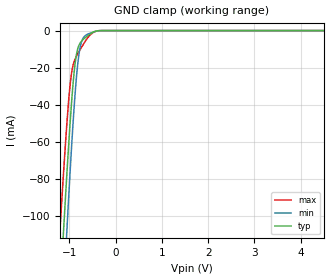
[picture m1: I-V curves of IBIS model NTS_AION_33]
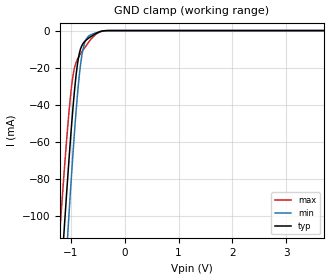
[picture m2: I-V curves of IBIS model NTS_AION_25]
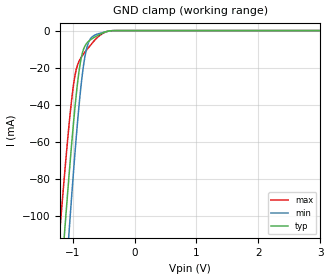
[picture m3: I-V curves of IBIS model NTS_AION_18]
| NXP Semiconductors
| Logic Products Group
| IBIS model of NTS0101
| SINGLE, DUAL-SUPPLY VOLTAGE-LEVEL TRANSLATING AUTO-DIRECTION SENSING
| TRANSCEIVER WITH OPEN-DRAIN OUTPUTS (3-STATE OE)
|[Packages]:
|[Package1]: SC88 (GW) 6-pin Package
|[Package2]: TSSOP6 (GV) 6-pins package
|[Package3]: XSON6 (GM) 6-pins package
|[Package4]: XSON6 (GF) 6-pins package
|[Package5]: XSON6 (GS) 6-pins package
[IBIS Ver]   3.2
[File Name]   nts0101.ibs
[File Rev]   1.0
[Date]   20-May-2011
[Source]   File created from simulations by LPG
   NXP Semiconductors Nijmegen
[Notes]   V1.0   Ibis model.
   Revision History
   Version Date   Author/Editor   Description
   1.0   May 2011   RRV   Initial Model
   Remarks: - The Power Clamp curves have been omitted from the input
   since there is no power clamp diode.
   - IBISCHK 5.0.3 used
[Disclaimer]
   NXP Semiconductors warrants and represents that the IBIS model
   identified herein is owned by NXP Semiconductors (NXP). The
   model provided is not warranted as fully representing all of the
   operating characteristics and specifications of the semiconductor
   products to which the model relates.  Moreover, unless there is a
   signed, written agreement to the contrary, this IBIS model is
   furnished on an "as is" basis without support or warranty of any
   kind, either expressed or implied, regarding the use thereof, and
   NXP specifically disclaims all implied warranties of
   merchantability and fitness of the model for any purpose.
   NXP does not assume any liability arising out of the application
   or use of this IBIS model including infringement of patents and
   copyrights, nor does NXP convey any license under its patents and
   copyrights or the rights of others.
   NXP provides IBIS models as a service to our customers. You and
   your company shall not distribute, convey, sell, or give these models
   to anyone else without receiving prior written permission from
   NXP.
   NXP reserves the right to make changes without notice to these
   IBIS models to improve reliability, function, or design.
   Please be aware that your receipt and subsequent use of the IBIS
   information provided shall serve as acceptance of the terms and
   conditions of this agreement.  If you do not accept these terms,
   you should return or destroy the IBIS models and any other
   accompanying information immediately.
[Copyright]
   (C) Copyright 2011 NXP Semiconductors
   All rights reserved
|   Info for  SC88 (GW) 6-pin Package
[Component]   NTS0101_GW
[Manufacturer]   NXP Semiconductors
[package]
|   typ   min   max
R_pkg  3.9397E-02  2.6064E-02  5.8029E-02
L_pkg  9.0534E-10  7.0046E-10  1.1872E-09
C_pkg  1.8035E-13  1.2290E-13  3.5012E-13
[Pin] signal_name   model_name   R_pin   L_pin   C_pin
   1   VDDA   POWER 3.0056E-02 7.6713E-10 1.2290E-13
   2   GND   GND 2.6064E-02 7.0046E-10 3.5012E-13
   3   A   NTS_AION 5.0072E-02 1.0663E-09 1.4645E-13
   4   B   NTS_BION 5.8029E-02 1.1872E-09 1.6820E-13
   5   OE   NTS_CTRLIN 3.4118E-02 8.2339E-10 1.5073E-13
   6   VDDB   POWER 3.8045E-02 8.8757E-10 1.4368E-13
|   Info for  TSSOP6 (GV) 6-pins package
[Component]   NTS0101_GV
[Manufacturer]   NXP Semiconductors
[Package]
|   Typ   Min   Max
R_pkg   8.223E-02   8.127E-02   8.329E-02
L_pkg   1.527E-09   1.437E-09   1.626E-09
C_pkg   2.754E-13   2.307E-13   4.138E-13
[Pin] signal_name   model_name   R_pin   L_pin   C_pin
   1   VDDA   POWER 8.329E-02 1.622E-09 2.613E-13
   2   GND   GND 8.127E-02 1.437E-09 4.138E-13
   3   A   NTS_AION 8.324E-02 1.626E-09 2.540E-13
   4   B   NTS_BION 8.183E-02 1.491E-09 2.307E-13
   5   OE   NTS_CTRLIN 8.187E-02 1.489E-09 2.619E-13
   6   VDDB   POWER 8.320E-02 1.613E-09 2.601E-13
|   Info for  XSON6 (GM) 6-pins package
[Component]   NTS0101_GM
[Manufacturer]   NXP Semiconductors
[Package]
|   Typ   Min   Max
R_pkg   3.997E-02   3.996E-02   3.998E-02
L_pkg   6.173E-10   6.152E-10   6.184E-10
C_pkg   1.884E-13   1.795E-13   2.057E-13
[Pin] signal_name   model_name   R_pin   L_pin   C_pin
   1   VDDA   POWER 3.997E-02 6.184E-10 1.801E-13
   2   GND   GND 3.996E-02 6.152E-10 2.057E-13
   3   A   NTS_AION 3.997E-02 6.182E-10 1.795E-13
   4   B   NTS_BION 3.998E-02 6.184E-10 1.795E-13
   5   OE   NTS_CTRLIN 3.997E-02 6.154E-10 2.057E-13
   6   VDDB   POWER 3.997E-02 6.179E-10 1.798E-13
|   Info for  XSON6 (GF) 6-pins package
[Component]   NTS0101_GF
[Manufacturer]   NXP Semiconductors
[Package]
|   Typ   Min   Max
R_pkg   3.978E-02   3.977E-02   3.979E-02
L_pkg   6.070E-10   6.066E-10   6.077E-10
C_pkg   1.209E-13   1.153E-13   1.316E-13
[Pin] signal_name   model_name   R_pin   L_pin   C_pin
   1   VDDA   POWER 3.979E-02 6.077E-10 1.160E-13
   2   GND   GND 3.979E-02 6.071E-10 1.316E-13
   3   A   NTS_AION 3.978E-02 6.072E-10 1.153E-13
   4   B   NTS_BION 3.977E-02 6.067E-10 1.153E-13
   5   OE   NTS_CTRLIN 3.978E-02 6.066E-10 1.315E-13
   6   VDDB   POWER 3.978E-02 6.069E-10 1.155E-13
|   Info for  XSON6 (GS) 6-pins package
[Component]   NTS0101_GS
[Manufacturer]   NXP Semiconductors
[Package]
|   Typ   Min   Max
R_pkg   3.5879E-02   3.5869E-02   3.5886E-02
L_pkg   4.5703E-10   4.5658E-10   4.5769E-10
C_pkg   1.1638E-13   1.1080E-13   1.2708E-13
[Pin] signal_name   model_name   R_pin   L_pin   C_pin
   1   VDDA   POWER 3.5886E-02 4.5769E-10 1.1155E-13
   2   GND   GND 3.5886E-02 4.5710E-10 1.2708E-13
   3   A   NTS_AION 3.5877E-02 4.5721E-10 1.1080E-13
   4   B   NTS_BION 3.5869E-02 4.5673E-10 1.1080E-13
   5   OE   NTS_CTRLIN 3.5878E-02 4.5658E-10 1.2704E-13
   6   VDDB   POWER 3.5879E-02 4.5686E-10 1.1098E-13
[Model Selector]   NTS_AION
NTS_AION_33   3.3V Vcc I/O model, non-inverting
NTS_AION_25   2.5V Vcc I/O model, non-inverting
NTS_AION_18   1.8V Vcc I/O model, non-inverting
[Model Selector]   NTS_BION
NTS_BION_50   5.0V Vcc I/O model, non-inverting
NTS_BION_33   3.3V Vcc I/O model, non-inverting
NTS_BION_25   2.5V Vcc I/O model, non-inverting
[Model Selector]   NTS_CTRLIN
NTS_CTRLIN_33   3.3V Vcc Input model
NTS_CTRLIN_25   2.5V Vcc Input model
NTS_CTRLIN_18   1.8V Vcc Input model
| Models and submodels in the file (9): NTS_AION_33 (Input), NTS_AION_25 (Input), NTS_AION_18 (Input), NTS_BION_50 (Input), NTS_BION_33 (Input), NTS_BION_25 (Input), NTS_CTRLIN_33 (Input), NTS_CTRLIN_25 (Input), NTS_CTRLIN_18 (Input)
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| Remark: If your software does not support the Model Selector
|   Please comment out the lines of the Model Selector, which
|   contain the name of the Model, except the one you want to use.
|   Model NTS_AION_33
[Model]   NTS_AION_33
Model_type   Input
Vinh  =  2.9
Vinl  =  0.15
C_comp   1.9335pF   1.4778pF   2.7541pF
[Model Spec]
| Note: The input and output voltage ratings may be exceeded if the input and
|   output current ratings are observed (please refer to the data sheet)
|   Subparameter   typ   min   max
Vinh   2.9   2.6   3.2
Vinl   0.15   0.15   0.15
| Overshoot
S_overshoot_high   6.5   6.5   6.5   | Static overshoot
S_overshoot_low   -0.5   -0.5   -0.5
D_overshoot_high   7.2   7.2   7.2   | Dynamic overshoot
D_overshoot_low   -1.0   -1.0   -1.0
D_overshoot_time   3n   3n   3n
|Ambient temperature:   25   85   -40
[Temperature Range]   40   100   -25
[Voltage Range]   3.3   3.0   3.6
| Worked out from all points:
|   GND clamp passes 1 mA (typ) near -0.50 V on its own axis
|Process Range   nominal   slow   fast
[GND_clamp]
|   voltage   I(typ)   I(min)   I(max)
-5.5V     -2.251A    -2.513A    -2.036A
-1.2V     -140.4mA   -178.4mA   -105.8mA
-1.12V    -105mA     -138.9mA   -74.04mA
-1.06V    -79.44mA   -110.2mA   -51.97mA
-1V       -55.52mA   -82.82mA   -33.13mA
-960mV    -41.02mA   -65.56mA   -24.03mA
-880mV    -18.45mA   -35.09mA   -15.56mA
-820mV    -9.803mA   -18.09mA   -12.49mA
-740mV    -5.756mA   -6.204mA   -9.073mA
-580mV    -2.41mA    -1.672mA   -3.148mA
-320mV    -16.74uA   -24.95uA   -12.41uA
5.5V      0A         0A         0A
|   Model NTS_AION_25
[Model]   NTS_AION_25
Model_type   Input
Vinh  =  2.1
Vinl  =  0.15
C_comp   1.9580pF   1.5348pF   2.7364pF
[Model Spec]
| Note: The input and output voltage ratings may be exceeded if the input and
|   output current ratings are observed (please refer to the data sheet)
|   Subparameter   typ   min   max
Vinh   2.1   1.9   2.3
Vinl   0.15   0.15   0.15
| Overshoot
S_overshoot_high   6.5   6.5   6.5   | Static overshoot
S_overshoot_low   -0.5   -0.5   -0.5
D_overshoot_high   7.2   7.2   7.2   | Dynamic overshoot
D_overshoot_low   -1.0   -1.0   -1.0
D_overshoot_time   3n   3n   3n
|Ambient temperature:   25   85   -40
[Temperature Range]   35   95   -35
[Voltage Range]   2.5   2.3   2.7
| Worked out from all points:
|   GND clamp passes 1 mA (typ) near -0.50 V on its own axis
|Process Range   nominal   slow   fast
[GND_clamp]
|   voltage   I(typ)   I(min)   I(max)
-5.5V     -2.251A    -2.513A    -2.036A
-1.2V     -140.4mA   -178.4mA   -105.8mA
-1.12V    -105mA     -138.9mA   -74.04mA
-1.06V    -79.44mA   -110.2mA   -51.97mA
-1V       -55.52mA   -82.82mA   -33.13mA
-960mV    -41.02mA   -65.56mA   -24.03mA
-880mV    -18.45mA   -35.09mA   -15.56mA
-820mV    -9.803mA   -18.09mA   -12.49mA
-740mV    -5.756mA   -6.204mA   -9.073mA
-580mV    -2.41mA    -1.672mA   -3.148mA
-320mV    -16.74uA   -24.95uA   -12.41uA
5.5V      0A         0A         0A
|   Model NTS_AION_18
[Model]   NTS_AION_18
Model_type   Input
Vinh  =  1.6
Vinl  =  0.15
C_comp   1.9936pF   1.6007pF   2.7364pF
[Model Spec]
| Note: The input and output voltage ratings may be exceeded if the input and
|   output current ratings are observed (please refer to the data sheet)
|   Subparameter   typ   min   max
Vinh   1.6   1.45   1.75
Vinl   0.15   0.15   0.15
| Overshoot
S_overshoot_high   6.5   6.5   6.5   | Static overshoot
S_overshoot_low   -0.5   -0.5   -0.5
D_overshoot_high   7.2   7.2   7.2   | Dynamic overshoot
D_overshoot_low   -1.0   -1.0   -1.0
D_overshoot_time   3n   3n   3n
|Ambient temperature:   25   85   -40
[Temperature Range]   35   95   -35
[Voltage Range]   1.8   1.65   1.95
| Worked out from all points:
|   GND clamp passes 1 mA (typ) near -0.50 V on its own axis
|Process Range   nominal   slow   fast
[GND_clamp]
|   voltage   I(typ)   I(min)   I(max)
-5.5V     -2.251A    -2.513A    -2.036A
-1.2V     -140.4mA   -178.4mA   -105.8mA
-1.12V    -105mA     -138.9mA   -74.04mA
-1.06V    -79.44mA   -110.2mA   -51.97mA
-1V       -55.52mA   -82.82mA   -33.13mA
-960mV    -41.02mA   -65.56mA   -24.03mA
-880mV    -18.45mA   -35.09mA   -15.56mA
-820mV    -9.803mA   -18.09mA   -12.49mA
-740mV    -5.756mA   -6.204mA   -9.073mA
-580mV    -2.41mA    -1.672mA   -3.148mA
-320mV    -16.74uA   -24.95uA   -12.41uA
5.5V      0A         0A         0A
